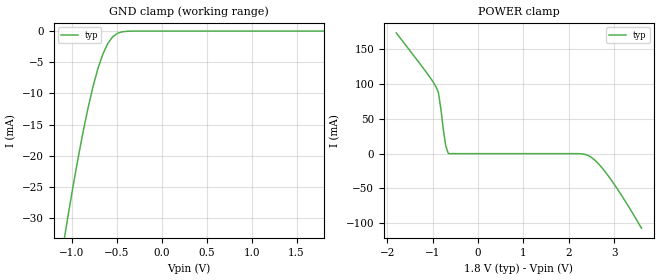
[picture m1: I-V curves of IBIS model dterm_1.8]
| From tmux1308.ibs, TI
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| dterm_1.8
[Model]   dterm_1.8
Model_type   Terminator
|   typ   min   max
C_comp   4.014581e-12   NA   NA
[Voltage Range]   1.8   NA   NA
[Temperature Range]   27   NA   NA
[Power Clamp Reference]   1.8   NA   NA
[GND Clamp Reference]   0   NA   NA
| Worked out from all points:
|   GND clamp passes 1 mA (typ) near -0.55 V on its own axis
|   POWER clamp passes 1 mA (typ) near -0.66 V on its own axis
[GND Clamp]
|   Voltage   I(typ)   I(min)   I(max)
-3.6V     -4.477kA   NA         NA
-1.091V   -34mA      NA         NA
-1.036V   -29.18mA   NA         NA
-872.7mV  -16.05mA   NA         NA
-763.6mV  -8.886mA   NA         NA
-709.1mV  -6.001mA   NA         NA
-654.5mV  -3.695mA   NA         NA
-600mV    -2.004mA   NA         NA
-545.5mV  -916.9uA   NA         NA
-436.4mV  -108.6uA   NA         NA
-327.3mV  -6.777uA   NA         NA
1.8V      873.5pA    NA         NA
[POWER Clamp]
|   Voltage   I(typ)   I(min)   I(max)
-1.8V     173.8mA    NA         NA
-1.091V   112.8mA    NA         NA
-872.7mV  88.34mA    NA         NA
-818.2mV  64.44mA    NA         NA
-763.6mV  34.53mA    NA         NA
-709.1mV  10.82mA    NA         NA
-654.5mV  296.5uA    NA         NA
2.4V      -2.004mA   NA         NA
2.618V    -12.27mA   NA         NA
2.836V    -29.18mA   NA         NA
3.164V    -60.32mA   NA         NA
3.6V      -107.2mA   NA         NA
